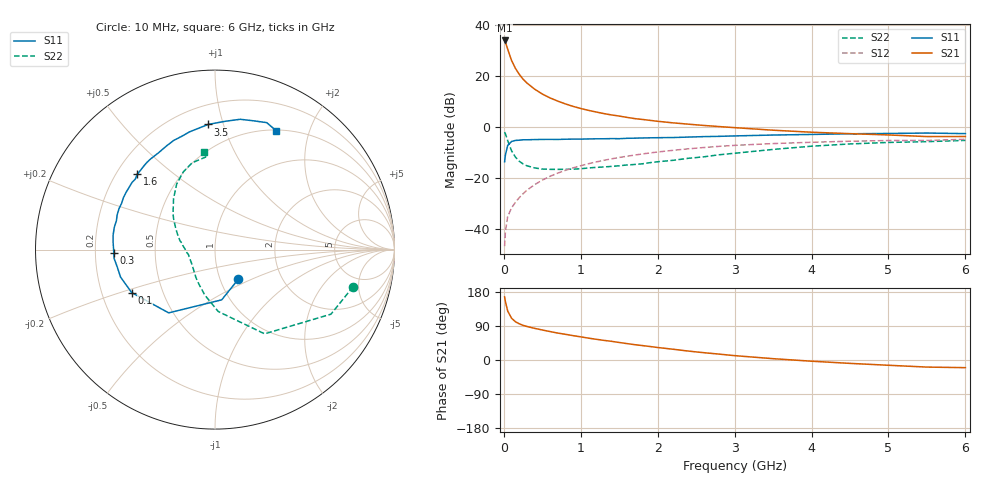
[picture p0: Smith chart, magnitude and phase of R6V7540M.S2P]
! SIEMENS Small Signal Semiconductors
! BFR193
! Si NPN RF Bipolar Junction Transistor in SOT23
! VCE = 0.75 V  IC = 40 mA
! Common Emitter S-Parameters:  May  1996
# GHz  S  MA  R  50
!  f  S11  S21  S12  S22
! GHz  MAG  ANG  MAG  ANG  MAG  ANG  MAG  ANG
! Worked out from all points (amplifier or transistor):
!   36 points, 10 MHz to 6 GHz, reference 50 ohm
!   highest |S21| = 33.9 dB at 10 MHz (marker M1)
!   |S21| within 3 dB of that: start of sweep to 45.64 MHz
!   unconditionally stable (mu >= 1): 258.9 MHz to 2.583 GHz; 5.609 GHz to end of sweep
!   at 250 MHz: K = 1.00, MSG = 22.4 dB, |S12| = -26.1 dB
!   at 1.4 GHz: K = 1.05, MAG = 7.2 dB, |S12| = -12.4 dB
!   at 6 GHz: K = 1.01, MAG = 0.1 dB, |S12| = -4.8 dB
!   S11 on the Smith chart (normalised r, x): 10 MHz: 1.22, -0.42; 100 MHz: 0.33, -0.22; 300 MHz: 0.28, -0.01; 1.6 GHz: 0.29, +0.38; 3.5 GHz: 0.33, +0.89; 6 GHz: 0.51, +1.52
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0.01  0.2101 -51.9  49.28 166.5  0.0047 75.5  0.797 -15.0
0.02  0.2824 -82.4  46.05 154.3  0.009 71.4  0.7396 -29.1
0.05  0.4368 -126.2  33.28 129.3  0.0179 61.0  0.5446 -59.5
0.1  0.5224 -152.7  20.11 110.3  0.0263 61.1  0.3453 -87.0
0.15  0.5481 -163.8  14.09 101.1  0.0337 63.4  0.2597 -102.6
0.2  0.5537 -170.3  10.76 95.5  0.0417 66.5  0.2151 -114.0
0.25  0.5643 -175.0  8.622 91.5  0.0497 68.0  0.1903 -123.6
0.3  0.5641 -178.3  7.274 88.5  0.0584 69.3  0.175 -130.1
0.4  0.5693 175.8  5.51 83.5  0.0749 70.2  0.1591 -140.5
0.5  0.5734 171.8  4.422 79.2  0.0918 70.3  0.1512 -149.7
0.6  0.5746 167.5  3.715 75.1  0.1089 69.6  0.1492 -155.7
0.7  0.5725 163.7  3.22 71.1  0.1257 68.8  0.1488 -160.0
0.8  0.5785 160.4  2.835 67.8  0.1426 67.3  0.1497 -164.5
0.9  0.5813 157.0  2.536 64.3  0.1593 66.1  0.1501 -168.5
1.1  0.5864 150.6  2.12 57.7  0.1922 63.1  0.1588 -174.4
1.6  0.6033 135.9  1.546 43.3  0.2687 54.7  0.1817 172.3
2.2  0.6241 120.4  1.208 28.4  0.3514 44.2  0.2238 158.3
2.8  0.6584 106.1  1.022 15.5  0.42 33.7  0.2877 143.3
3.5  0.6984 93.1  0.868 3.5  0.4756 22.0  0.3655 129.2
4.5  0.7397 79.0  0.743 -8.9  0.5287 8.0  0.468 112.1
5.5  0.7639 67.8  0.652 -18.7  0.5476 -4.7  0.5183 95.7
6  0.7443 62.7  0.654 -20.2  0.5768 -8.7  0.5488 96.7
